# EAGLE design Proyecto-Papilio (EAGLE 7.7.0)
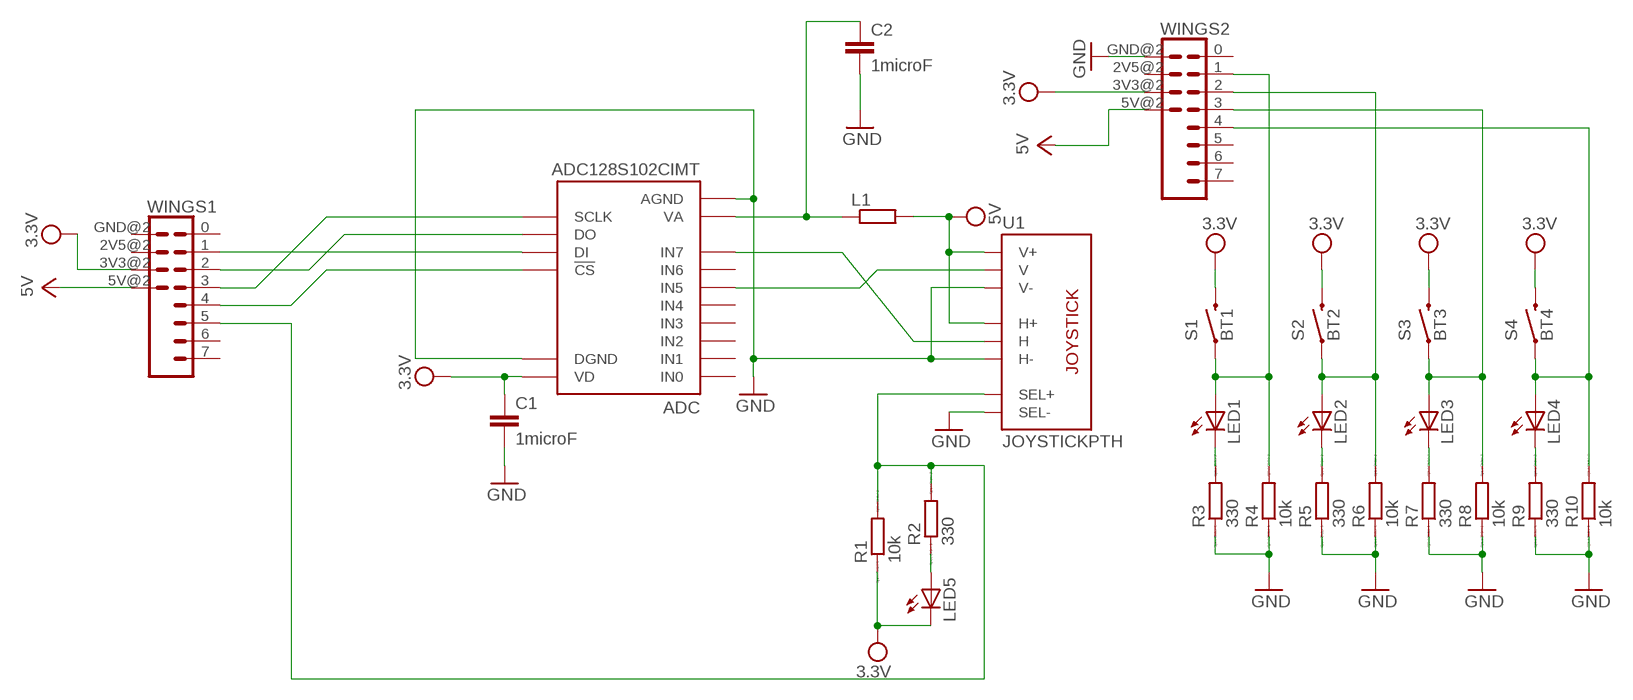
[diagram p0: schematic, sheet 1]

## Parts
ADC  ADC128S102CIMT  [TSSOP16]
C1  1microF  C-EUC0805  [C0805]
C2  1microF  C-EUC0805  [C0805]
L1  R-EU_R0805  [R0805]
LED1  LED3MM  [LED3MM]
LED2  LED3MM  [LED3MM]
LED3  LED3MM  [LED3MM]
LED4  LED3MM  [LED3MM]
LED5  LED3MM  [LED3MM]
R1  10k  RR1206  [R1206]
R2  330  RR1206  [R1206]
R3  330  RR1206  [R1206]
R4  10k  RR1206  [R1206]
R5  330  RR1206  [R1206]
R6  10k  RR1206  [R1206]
R7  330  RR1206  [R1206]
R8  10k  RR1206  [R1206]
R9  330  RR1206  [R1206]
R10  10k  RR1206  [R1206]
S1  BT1  SWITCH-MOMENTARY-212MM  [TACTILE-PTH-12MM]
S2  BT2  SWITCH-MOMENTARY-212MM  [TACTILE-PTH-12MM]
S3  BT3  SWITCH-MOMENTARY-212MM  [TACTILE-PTH-12MM]
S4  BT4  SWITCH-MOMENTARY-212MM  [TACTILE-PTH-12MM]
U1  JOYSTICKPTH  [JOYSTICK]
WINGS1  WING8  WING8WING8_NOHOLES  [WINGSIDE_8BIT_NOHOLES]
WINGS2  WING8  WING8WING8_NOHOLES  [WINGSIDE_8BIT_NOHOLES]

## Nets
GND: ADC.3(AGND) ADC.12(DGND) C1.2 C2.2 R3.1 R4.1 R5.1 R6.1 R7.1 R8.1 R9.1 R10.1 U1.B2A(SEL-) U1.H3(H-) U1.V3(V-) WINGS2.GND@2(GND)
N$1: ADC.14(DI) WINGS1.1
N$2: ADC.15(DO) WINGS1.2
N$3: LED4.A R10.2 S4.1 WINGS2.4
N$4: ADC.16(SCLK) WINGS1.3
N$5: ADC.1(!CS) WINGS1.4
N$6: LED5.A R2.1
N$7: ADC.11(IN7) U1.H2(H)
N$9: ADC.9(IN5) U1.V2(V)
N$11: R1.2 R2.2 U1.B1A(SEL+) WINGS1.5
N$13: LED2.A R6.2 S2.1 WINGS2.2
N$16: LED2.K(C) R5.2
N$17: LED1.A R4.2 S1.1 WINGS2.1
N$18: LED1.K(C) R3.2
N$25: LED3.K(C) R7.2
N$26: LED3.A R8.2 S3.1 WINGS2.3
N$30: LED4.K(C) R9.2
V+: WINGS1.5V@2(5V) WINGS2.5V@2(5V) ; supply symbol labelled 5V
VA: ADC.2(VA) C2.1 L1.1
VDD: ADC.13(VD) C1.1 L1.2 LED5.K(C) R1.1 S1.3 S2.3 S3.3 S4.3 U1.H1(H+) U1.V1(V+) WINGS1.3V3@2(3V3) WINGS2.3V3@2(3V3) ; supply symbol labelled 3.3V, 5V
Unconnected: ADC.4(IN0) ADC.5(IN1) ADC.6(IN2) ADC.7(IN3) ADC.8(IN4) ADC.10(IN6) WINGS1.0 WINGS1.2V5@2(2V5) WINGS1.6 WINGS1.7 WINGS1.GND@2(GND) WINGS2.0 WINGS2.2V5@2(2V5) WINGS2.5 WINGS2.6 WINGS2.7

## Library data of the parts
ADC = bt_adc:ADC128S: ADC128S102 The ADC128S102 is a low-power, eight-channel CMOS 12- bit analog-to-digital converter specified for conversion throughput rates of 500 ksps to 1 MSPS, featuring output serial data that is straight binary and is compatible with several standards, such as SPI?, QSPI?, MICROWIRE?, and many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
C1 C2 = resistor:C-EU: CAPACITOR, European symbol
L1 = resistor:R-EU_: RESISTOR, European symbol
LED1-LED5 = adafruit:LED: LED
R1-R10 = eagle-ltspice:R: RESISTOR, European symbol; SPICEMODEL: NONE; SPICEPREFIX: R
S1-S4 = SparkFun-Electromechanical:SWITCH-MOMENTARY-2: Various NO switches- pushbuttons, reed, etc; PROD_ID: SWCH-09185
U1 = SparkFun-Electromechanical:JOYSTICK: Thumb Joystick Joystick commonly found in PS2 controllers. Two pots and a select switch. Footprint proven. Spark Fun Electronics SKU : COM-09032
WINGS1 WINGS2 = Papilio:WING8

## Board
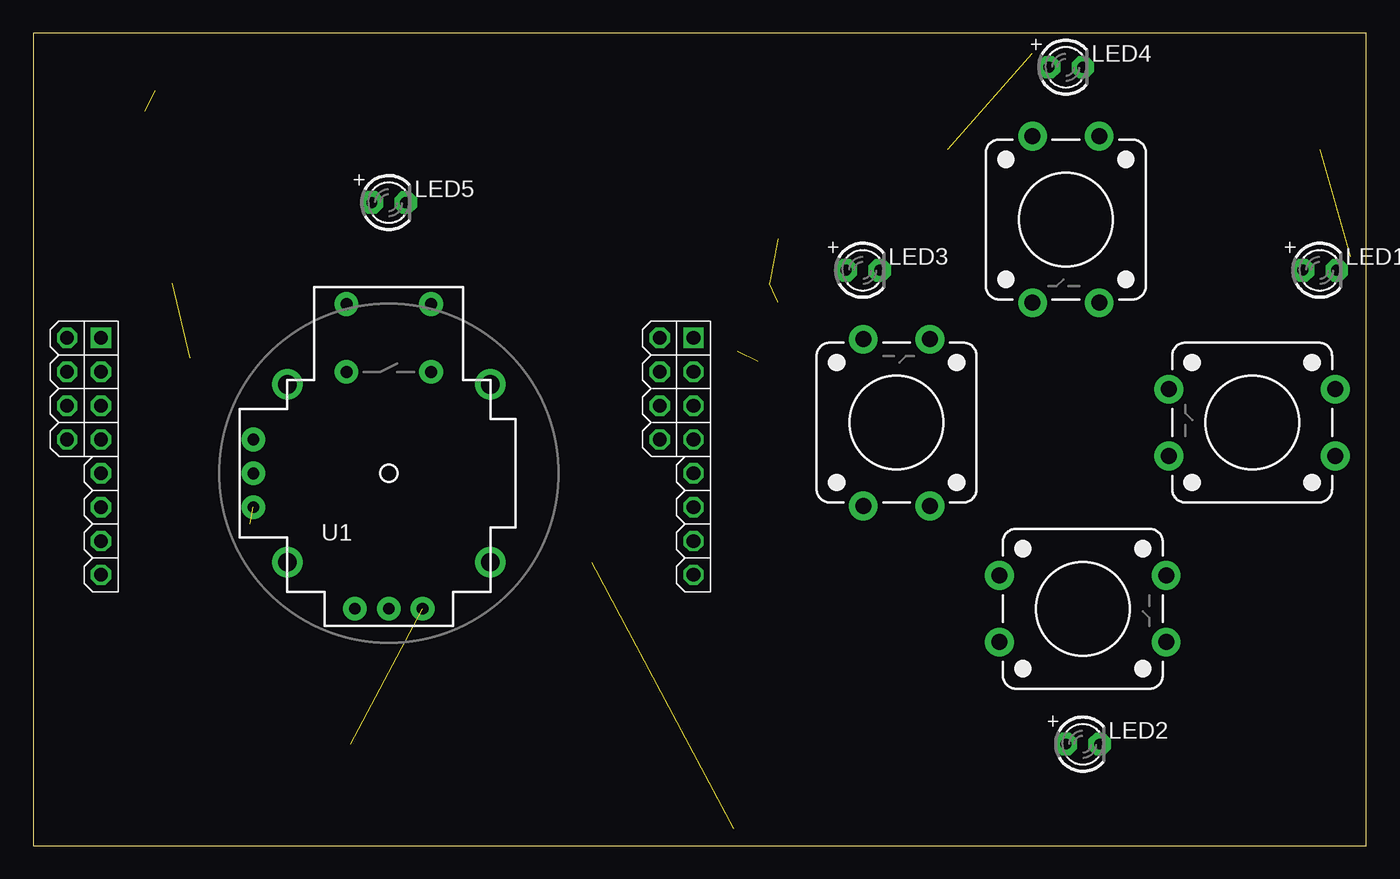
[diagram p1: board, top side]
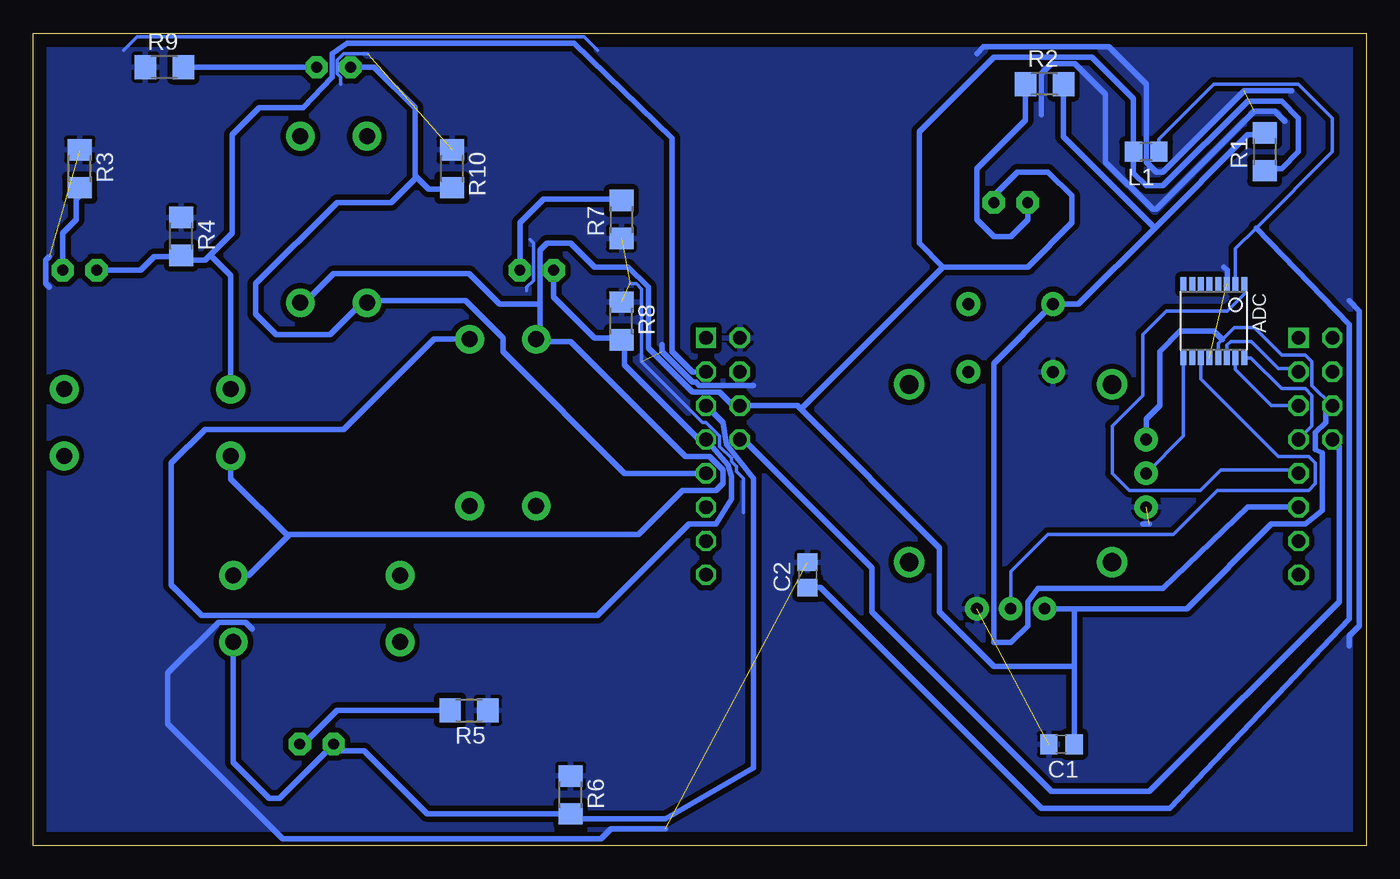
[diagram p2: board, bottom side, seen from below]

Size 100 x 60.95 mm. Coordinates in mm from the lower left corner, seen from the top.
Outline: 0,0 100,0 100,60.95 0,60.95 0,0
Copper layers (1*16): Top 0.035mm / dielectric 1.5mm / Bottom 0.035mm
Design rules "default": minimum track width 10mil, minimum drill 24mil, track to track 8mil, track to pad 8mil, pad to pad 8mil, via to via 8mil, smd to smd 8mil, copper to edge 40mil, drill to drill 8mil, minimum pad ring 10mil, minimum via ring 8mil, stop-mask expansion 4mil, vias tented up to drill 0mil, thermal gap 10mil

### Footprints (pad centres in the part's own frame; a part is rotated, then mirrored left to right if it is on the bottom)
TSSOP16 = smd 0.45 x 1.05: 1 -2.275,-2.768; 2 -1.625,-2.768; 3 -0.975,-2.768; 4 -0.325,-2.768; 5 0.325,-2.768; 6 0.975,-2.768; 7 1.625,-2.768; 8 2.275,-2.768; 9 2.275,2.768; 10 1.625,2.768; 11 0.975,2.768; 12 0.325,2.768; 13 -0.325,2.768; 14 -0.975,2.768; 15 -1.625,2.768; 16 -2.275,2.768
C0805 = smd 1.3 x 1.5: 1 -0.95,0; 2 0.95,0
R0805 = smd 1.3 x 1.5: 1 -0.95,0; 2 0.95,0
LED3MM = drill 0.813 pad 1.676 octagon: A -1.27,0; K 1.27,0
R1206 = smd 1.6 x 1.803: 1 -1.422,0; 2 1.422,0
TACTILE-PTH-12MM = drill 1.2 pad 2.159: 1 6.25,-2.5; 2 -6.25,-2.5; 3 6.25,2.5; 4 -6.25,2.5
JOYSTICK = drill 0.9 pad 1.778: B1A -3.175,12.7; B1B 3.175,12.7; B2A -3.175,7.62; B2B 3.175,7.62 | drill 0.889 pad 1.778: H1 -2.54,-10.16; H2 0,-10.16; H3 2.54,-10.16; V1 -10.16,2.54; V2 -10.16,0; V3 -10.16,-2.54 | drill 1.397 pad 2.286: MOUNT1 -7.62,6.668; MOUNT2 -7.62,-6.668; MOUNT3 7.62,-6.668; MOUNT4 7.62,6.668
WINGSIDE_8BIT_NOHOLES = drill 1.016 square: 0 19.05,1.27 | drill 1.016 octagon: 1 16.51,1.27; 2 13.97,1.27; 2V5@2 16.51,3.81; 3 11.43,1.27; 3V3@2 13.97,3.81; 4 8.89,1.27; 5 6.35,1.27; 5V@2 11.43,3.81; 6 3.81,1.27; 7 1.27,1.27; GND@2 19.05,3.81

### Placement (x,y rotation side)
ADC  11.43,39.37 180 bottom
C1  22.86,7.62 180 bottom
C2  41.91,20.32 90 bottom
L1  16.51,52.07 180 bottom
LED1  96.52,43.18 0 top
LED2  78.74,7.62 0 top
LED3  62.23,43.18 0 top
LED4  77.47,58.42 0 top
LED5  26.67,48.26 0 top
R1  7.62,52.07 90 bottom
R2  24.13,57.15 0 bottom
R3  96.52,50.8 270 bottom
R4  88.9,45.72 270 bottom
R5  67.31,10.16 180 bottom
R6  59.69,3.81 270 bottom
R7  55.88,46.99 90 bottom
R8  55.88,39.37 270 bottom
R9  90.17,58.42 0 bottom
R10  68.58,50.8 270 bottom
S1  91.44,31.75 180 top
S2  78.74,17.78 0 top
S3  64.77,31.75 90 top
S4  77.47,46.99 270 top
U1  26.67,27.94 0 top
WINGS1  6.35,19.05 90 top
WINGS2  50.8,19.05 90 top

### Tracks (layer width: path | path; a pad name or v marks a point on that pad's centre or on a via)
GND  (11 unrouted)
  Bottom 0.254: 62.99,41.66 62.99,41.91 62.48,42.42 62.48,45.21 62.74,45.47 | 57.66,59.69 58.67,60.71 92.2,60.71 93.22,59.69 | 76.96,57.15 76.96,57.66 77.22,57.91 77.22,58.93 76.71,59.44 74.93,59.44 | 46.74,25.02 46.74,27.56 47.24,28.07 47.24,28.45 47.62,28.83 47.62,29.08 48.51,29.97 48.51,30.73 49.53,31.75 49.78,31.75 54.36,36.32 54.36,41.78 54.74,42.16 55.24,42.16
  Bottom 0.406: 52.58,1.27 56.64,1.27 57.4,0.51 81.28,0.51 89.92,9.14 89.92,12.95 86.11,16.76 84.07,16.76 83.57,16.26 | 5.59,56.64 9.14,56.64 15.24,50.55 15.75,50.55 16.51,51.31 16.51,57.15 19.3,59.94 28.7,59.94 29.21,59.44 | 24.38,54.86 24.38,57.91 23.62,58.67 21.84,58.67 19.56,56.39 19.56,51.31 16,47.75 15.75,47.75 8.38,55.12 6.86,55.12 6.1,54.36 | 98.81,44.2 99.06,43.94 99.06,42.16 98.81,41.91 | 1.27,14.99 1.27,15.75 0.51,16.51 0.51,40.13 1.27,40.89 | 16.26,24.13 16.76,24.13 | 10.41,42.16 10.41,43.18 10.67,43.43 | 52.83,37.59 52.83,37.08 50.55,34.8 50.29,34.8 50.04,34.54 45.97,34.54
  pour Bottom (isolate 0.406): 0,60.96 100.33,60.96 100.33,0 0,0
N$1
  Bottom 0.254: ADC.14 10.46,37.55 10.16,37.85 8.64,37.85 6.6,35.81 5.33,35.81 WINGS1.1
N$2
  Bottom 0.254: ADC.15 9.8,35.71 7.11,33.02 WINGS1.2
N$3
  Bottom 0.406: LED4.A 74.42,58.42 71.37,55.37 71.37,50.29 71.25,50.16 | 71.25,50.16 70.36,49.28 68.68,49.28 R10.2 | 71.25,50.16 73.15,48.26 77.22,48.26 83.31,42.16 83.31,39.88 81.79,38.35 77.72,38.35 75.34,40.74 S4.1 74.82,40.89 67.56,40.89 64.77,38.1 64.77,37.08 55.63,27.94 WINGS2.4
N$4
  Bottom 0.254: ADC.16 8.66,36.6 6.35,34.29 4.57,34.29 4.06,33.78 4.06,31.5 WINGS1.3
N$5
  Bottom 0.254: ADC.1 9.15,41.39 10.41,40.13 14.99,40.13 16.76,38.35 16.76,33.78 19.05,31.5 19.05,27.94 17.78,26.67 12.45,26.67 10.92,28.19 5.33,28.19 WINGS1.4
N$6
  Bottom 0.406: R2.1 25.55,54.46 29.21,50.8 29.21,46.99 27.94,45.72 26.67,45.72 25.4,46.99 LED5.A
N$7
  Bottom 0.254: ADC.11 12.4,35.01 6.6,29.21 4.32,29.21 3.81,28.7 3.81,27.18 4.32,26.67 11.18,26.67 14.48,23.37 23.88,23.37 26.67,20.57 U1.H2
N$9
  Bottom 0.254: ADC.9 13.71,30.75 U1.V2
N$11
  Bottom 0.406: 15.88,46.35 21.59,40.64 U1.B1A 27.94,36.2 27.94,15.24 26.67,15.24 25.4,16.51 25.4,18.29 24.64,19.3 15.24,19.3 8.89,25.4 WINGS1.5 | 15.88,46.35 8.89,53.34 7.77,53.34 R1.2 | R2.2 22.71,53.19 15.88,46.35
N$13
  Bottom 0.406: WINGS2.2 48.26,31.75 48.01,30.1 45.97,27.56 45.97,5.84 52.58,2.03 59.33,2.03 R6.2 70.46,2.39 75.18,7.11 76.96,7.11 LED2.A 81.53,3.56 82.3,3.56 84.99,6.25 S2.1
N$16
  Bottom 0.406: LED2.K 79.76,7.62 77.22,10.16 R5.2
N$17
  Bottom 0.406: WINGS2.1 50.55,35.56 52.07,37.08 52.07,53.09 59.44,60.2 76.45,60.2 77.6,59.44 77.6,57.66 79.76,55.37 83.06,55.37 85.09,53.34 85.09,45.97 86.74,44.32 | 86.74,44.32 87.12,43.94 88.54,43.94 R4.2 89,44.2 90.93,44.2 91.95,43.18 LED1.A | S1.1 85.19,42.77 86.74,44.32
N$18
  Bottom 0.406: LED1.K 97.79,45.97 96.77,46.99 96.77,48.51 96.52,48.77 R3.2
N$25
  Bottom 0.406: LED3.K 63.5,46.74 61.72,48.51 55.98,48.51 R7.2
N$26
  Bottom 0.406: LED3.A 60.96,41.15 57.91,38.1 56.03,38.1 R8.2 55.63,37.69 55.63,36.07 50.04,30.48 WINGS2.3 47.88,28.57 47.62,27.69 47.62,26.04 48.77,24.13 50.8,24.13 57.66,17.27 87.38,17.27 89.66,19.56 89.66,28.7 87.12,31.24 76.71,31.24 69.95,38 S3.1
N$30
  Bottom 0.406: LED4.K R9.2
V+
  Bottom 0.406: WINGS2.5V@2 46.74,30.48 37.08,20.83 37.08,17.53 23.62,4.06 16.26,4.06 2.03,18.29 2.03,29.97 WINGS1.5V@2
VA
  Bottom 0.254: L1.1 15.56,53.02 11.43,57.15 5.08,57.15 2.54,54.61 2.54,52.07 8.26,46.35 9.8,44.8 ADC.2
  Bottom 0.406: C2.1 40.96,19.37 24.38,2.79 14.73,2.79 1.27,17.02 1.27,39.12 8.26,46.35
VDD
  Bottom 0.254: ADC.13 11.11,37.66 10.79,37.97 9.91,38.86 8.38,38.86 6.35,36.83 4.57,36.83 4.06,36.32 4.06,34.54 WINGS1.3V3@2
  Bottom 0.406: R1.1 7.47,50.8 6.35,50.8 5.08,52.07 5.08,54.61 6.35,55.88 8.89,55.88 15.24,49.53 16.51,49.53 17.46,50.48 L1.2 17.46,56.07 20.57,59.18 27.94,59.18 33.53,53.59 33.53,45.21 31.75,43.43 | U1.H1 21.84,17.78 | 21.84,17.78 13.46,17.78 7.11,24.13 4.57,24.13 3.3,25.15 3.3,29.46 3.81,29.72 3.81,30.99 3.05,31.75 3.05,32.51 WINGS1.3V3@2 | C1.1 21.91,13.46 | 21.91,13.46 21.91,17.71 21.84,17.78 | 42.42,32.77 42.67,33.02 WINGS2.3V3@2 47.5,33.02 48.51,34.04 50.55,34.04 53.85,37.34 53.85,41.91 55.37,43.43 57.91,43.43 59.69,45.21 61.47,45.21 61.98,44.7 61.98,40.64 | 42.42,32.77 32,22.35 32,17.53 27.94,13.46 21.91,13.46 | LED5.K 27.94,48.77 26.16,50.55 23.88,50.55 22.1,48.77 22.1,46.74 25.4,43.43 31.75,43.43 | 31.75,43.43 42.42,32.77 | U1.V1 16.51,32 15.49,33.02 15.49,37.08 13.97,38.61 11.43,38.61 10.79,37.97 | 61.98,40.64 61.98,38.04 S3.3 62.12,37.85 59.69,37.85 51.05,29.21 49.28,29.21 48.26,28.19 48.26,27.18 48.77,26.67 51.31,26.67 54.61,23.37 80.77,23.37 80.9,23.24 | S4.3 79.66,40.74 77.47,42.93 67.31,42.93 65.02,40.64 61.98,40.64 | S2.3 83.86,20.28 80.9,23.24 | S1.3 85.19,27.53 80.9,23.24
